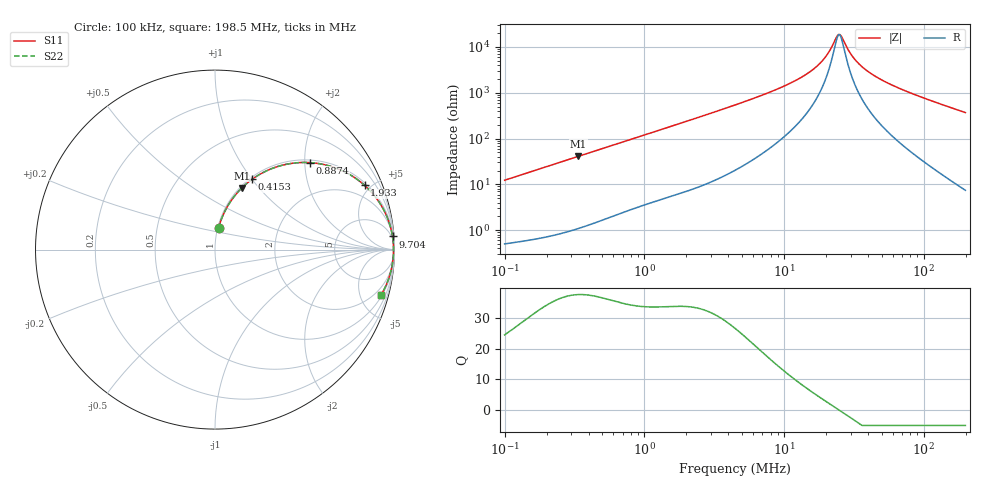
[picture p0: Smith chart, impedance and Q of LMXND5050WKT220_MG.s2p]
! LMXND5050WKT220_MG  S-PARAMETER MODEL  ( General Type )
! Model Generated by TAIYO YUDEN Corporation (http://www.ty-top.com)
! Version 1.0
! TAIYO YUDEN Control No. 191023NI43SB-FBB
! Copyright(c) 2019 TAIYO YUDEN CO.,LTD. All Rights Reserved.
! Product Description (link to TY-COMPAS)
! https://ds.yuden.co.jp/TYCOMPAS/or/detail?pn=LMXND5050WKT220MMG&u=M
! Products Name : Inductors
! Characteristics :
!  Inductance : 22 uH , SRF(min) : 17 MHz , DC Resistance(max) : 0.312 Ohm
!  Rated Current : Saturation :900 mA , Temp Rise : 1000 mA
!  Case Size : 4.9 x 4.9 / 0.193 x 0.193 [mm/inch] , Thickness : 2 / 0.079 [mm/inch]
!  (Conditions: Temperature = 25 degC , DC Bias Current/Voltage = 0A / 0V)
! External Node Assignments :
!  1  o---GGG---o  2
! GND o---------o GND
! Frequency Range : 0.1MHz  -  198.534594MHz  [ 402 STEP ]
# MHz S RI R 50
! Freq[MHz].  S11 Real  S11 Imag  S21 Real  S21 Imag  S12 Real  S12 Imag  S22 Real  S22 Imag
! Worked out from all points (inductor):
!   401 points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, 100 kHz to 198.5 MHz, reference 50 ohm
!   read as one part in series: L = 19.5 uH near 103.9 kHz
!   highest Q = 37.7 at 337 kHz (marker M1), where L = 19.3 uH
!   self-resonance near 24.6 MHz
!   S11 on the Smith chart (normalised r, x): 100 kHz: 1.01, +0.25; 415.3 kHz: 1.03, +1.00; 887.4 kHz: 1.06, +2.12; 1.933 MHz: 1.14, +4.58; 9.704 MHz: 3, +27; 198.5 MHz: 1.15, -7.37
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0.1  0.0196 0.1197  0.9804 -0.1197  0.9804 -0.1197  0.0196 0.1197
0.20186  0.0629 0.2287  0.9371 -0.2287  0.9371 -0.2287  0.0629 0.2287
0.337019  0.1496 0.3437  0.8504 -0.3437  0.8504 -0.3437  0.1496 0.3437
0.356769  0.164 0.3573  0.836 -0.3573  0.836 -0.3573  0.164 0.3573
0.415283  0.2079 0.3926  0.7921 -0.3926  0.7921 -0.3926  0.2079 0.3926
0.887417  0.5291 0.4846  0.4709 -0.4846  0.4709 -0.4846  0.5291 0.4846
1.272844  0.6912 0.4474  0.3088 -0.4474  0.3088 -0.4474  0.6912 0.4474
1.932663  0.833 0.3585  0.167 -0.3585  0.167 -0.3585  0.833 0.3585
4.541117  0.9619 0.1734  0.0381 -0.1734  0.0381 -0.1734  0.9619 0.1734
9.7039  0.989 0.0733  0.011 -0.0733  0.011 -0.0733  0.989 0.0733
15.89665  0.9936 0.0313  0.00635 -0.0313  0.00635 -0.0313  0.9936 0.0313
19.21992  0.9944 0.0176  0.00563 -0.0176  0.00563 -0.0176  0.9944 0.0176
21.13365  0.9946 0.011  0.00543 -0.011  0.00543 -0.011  0.9946 0.011
23.68329  0.9947 0.00315  0.0053 -0.00315  0.0053 -0.00315  0.9947 0.00315
25.07124  0.9947 -0.000733  0.00529 0.000733  0.00529 0.000733  0.9947 -0.000733
26.04144  0.9947 -0.00332  0.00529 0.00332  0.00529 0.00332  0.9947 -0.00332
30.3125  0.9945 -0.0138  0.00546 0.0138  0.00546 0.0138  0.9945 -0.0138
34.62054  0.9942 -0.0231  0.0058 0.0231  0.0058 0.0231  0.9942 -0.0231
42.66034  0.9932 -0.0387  0.00677 0.0387  0.00677 0.0387  0.9932 -0.0387
56.71438  0.9908 -0.0628  0.00923 0.0628  0.00923 0.0628  0.9908 -0.0628
96.50321  0.9795 -0.1219  0.0205 0.1219  0.0205 0.1219  0.9795 -0.1219
198.5346  0.927 -0.2502  0.073 0.2502  0.073 0.2502  0.927 -0.2502
